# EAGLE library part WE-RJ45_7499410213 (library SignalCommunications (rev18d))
WE-RJ45 LAN Transformer Order Code 7499410213 Design THT xBase-T 10/100 Base-T Ports 1x1 Application Standard Tab Position DOWN LED (Left-Right) YELLOW-GREEN EMI Fingers No Details see: http://katalog.we-online.de/en/pbs/WE-LAN-RJ45 Created by Yingchun Shan 2016 (C) Wurth Elektronik
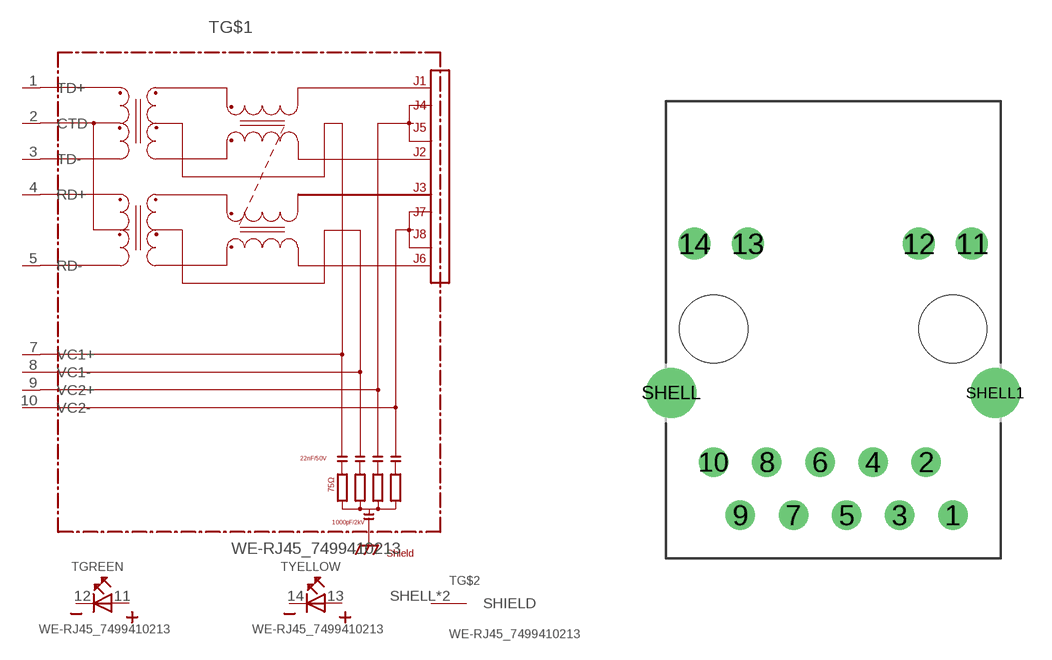
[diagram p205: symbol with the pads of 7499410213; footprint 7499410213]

Designator prefix T; gates G$1=7499410213 GREEN=LED_2PIN YELLOW=LED_2PIN G$2=SHIELD

## WE-RJ45_7499410213  [7499410213]
1  G$1:TD+
2  G$1:CTD
3  G$1:TD-
4  G$1:RD+
5  G$1:RD-
7  G$1:VC1+
8  G$1:VC1-
9  G$1:VC2+
10  G$1:VC2-
11  GREEN:A  pas
12  GREEN:K  pas
13  YELLOW:A  pas
14  YELLOW:K  pas
SHELL  G$2:SHIELD  pas
SHELL1  G$2:SHIELD  pas

## Footprint 7499410213 (pad centres in mm)
drill 0.9: 1 5.715,-8.89; 2 4.445,-6.35; 3 3.175,-8.89; 4 1.905,-6.35; 5 0.635,-8.89; 6 -0.635,-6.35; 7 -1.905,-8.89; 8 -3.175,-6.35; 9 -4.445,-8.89; 10 -5.715,-6.35
drill 1.02: 11 6.63,4.08; 12 4.09,4.08; 13 -4.09,4.08; 14 -6.63,4.08
drill 1.6: SHELL -7.745,-3.05; SHELL1 7.745,-3.05
hole 3.25 at -5.715,0
hole 3.25 at 5.715,0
